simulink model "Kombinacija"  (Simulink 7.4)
settings: Solver=FixedStepDiscrete  StartTime=0.0  StopTime=10.0  RelTol=1e-3
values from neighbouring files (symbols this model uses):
  A = [zeros(1,Ocenjeni_premik-1);[eye(Ocenjeni_premik-2),zeros(Ocenjeni_premik-2,1)]]    [Paprika.m]    (also in Primer_12_2.m = [0.1 0.6;-0.1 -0.4]; Primer_12_3.m = [0.1 0.6;-0.1 -0.4]; Primer_12_kombinacija.m = [0.1 0.6;-0.1 -0.4]; Liapunov_Linearni.m = [-0.5 0;0 -0.5])
  B = [1;zeros(Ocenjeni_premik-2,1)]    [Paprika.m]    (also in Primer_12_2.m = [0.3;0.1]; Primer_12_3.m = [0.3;0.1]; Primer_12_kombinacija.m = [0.3;0.1]; Primer_14_1.m = [0; 1])
  C = ones(1,Ocenjeni_premik-1)/(Ocenjeni_premik)    [Paprika.m]    (also in Primer_12_2.m = eye(2); Primer_12_3.m = [1 1]; Primer_12_kombinacija.m = [1 1]; Primer_14_1.m = [1 0])
  D = 1/(Ocenjeni_premik)    (= 0.0322580645161)    [Paprika.m]    (also in Primer_12_2.m = 0; Primer_12_3.m = 0; Primer_12_kombinacija.m = 0; Primer_14_1.m = 0)
  h = place(A.',C.',[0+1000000*eps 0-1000000*eps]).'    [Primer_12_3.m]    (also in Primer_12_kombinacija.m; Oversampling.m = figure; y_je_konv_u_g.m = dimpulse(Stevec,Imenovalec,h_os); OdzivInLastniVektorji.m = plot(x(1),x(2),'g*'))
  k = place(A,B,[0+1e4*eps 0-1e4*eps])    [Primer_12_2.m]    (also in Primer_12_kombinacija.m = place(A,B,[0+1000*eps 0-1000*eps]); Razs_z_transm.m = sym('k','positive'); Primer_14_2.m = sym('k','positive'))

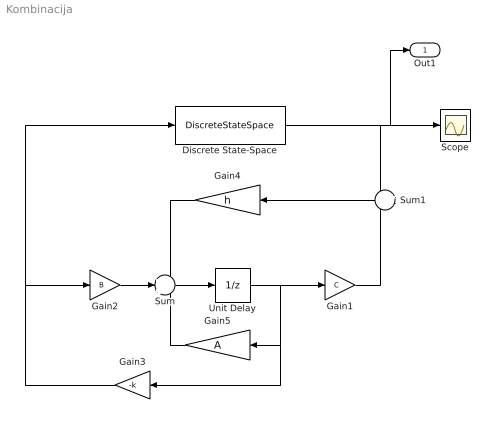
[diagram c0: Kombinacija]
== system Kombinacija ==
  Discrete State-Space : DiscreteStateSpace  A=A  B=B  C=C  D=D  X0=[1; 1]
  Gain1 : Gain  Gain=C  Multiplication=Matrix(K*u)  ParameterDataType=fixdt(1, 16)  ParameterScaling=2^0  OutDataType=fixdt(1, 16)  OutScaling=2^0
  Gain2 : Gain  Gain=B  Multiplication=Matrix(K*u)  ParameterDataType=fixdt(1, 16)  ParameterScaling=2^0  OutDataType=fixdt(1, 16)  OutScaling=2^0
  Gain3 : Gain  Gain=-k  Multiplication=Matrix(K*u)  ParameterDataType=fixdt(1, 16)  ParameterScaling=2^0  OutDataType=fixdt(1, 16)  OutScaling=2^0
  Gain4 : Gain  Gain=h  Multiplication=Matrix(K*u)  ParameterDataType=fixdt(1, 16)  ParameterScaling=2^0  OutDataType=fixdt(1, 16)  OutScaling=2^0
  Gain5 : Gain  Gain=A  Multiplication=Matrix(K*u)  ParameterDataType=fixdt(1, 16)  ParameterScaling=2^0  OutDataType=fixdt(1, 16)  OutScaling=2^0
  Scope : Scope
  Sum : Sum  Inputs=+++  OutDataType=fixdt(1, 16)  OutScaling=2^0
  Sum1 : Sum  Inputs=+-  OutDataType=fixdt(1, 16)  OutScaling=2^0
  Unit Delay : UnitDelay  X0=[0;0]  SampleTime=-1
  Out1 : Outport  OutDataType=fixdt(1, 16)  OutScaling=2^0
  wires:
  Unit Delay/1 -> Gain1/1, Gain5/1, Gain3/1
  Sum/1 -> Unit Delay/1
  Gain4/1 -> Sum/1
  Gain2/1 -> Sum/2
  Gain5/1 -> Sum/3
  Discrete State-Space/1 -> Sum1/1, Scope/1, Out1/1
  Gain1/1 -> Sum1/2
  Sum1/1 -> Gain4/1
  Gain3/1 -> Discrete State-Space/1, Gain2/1
